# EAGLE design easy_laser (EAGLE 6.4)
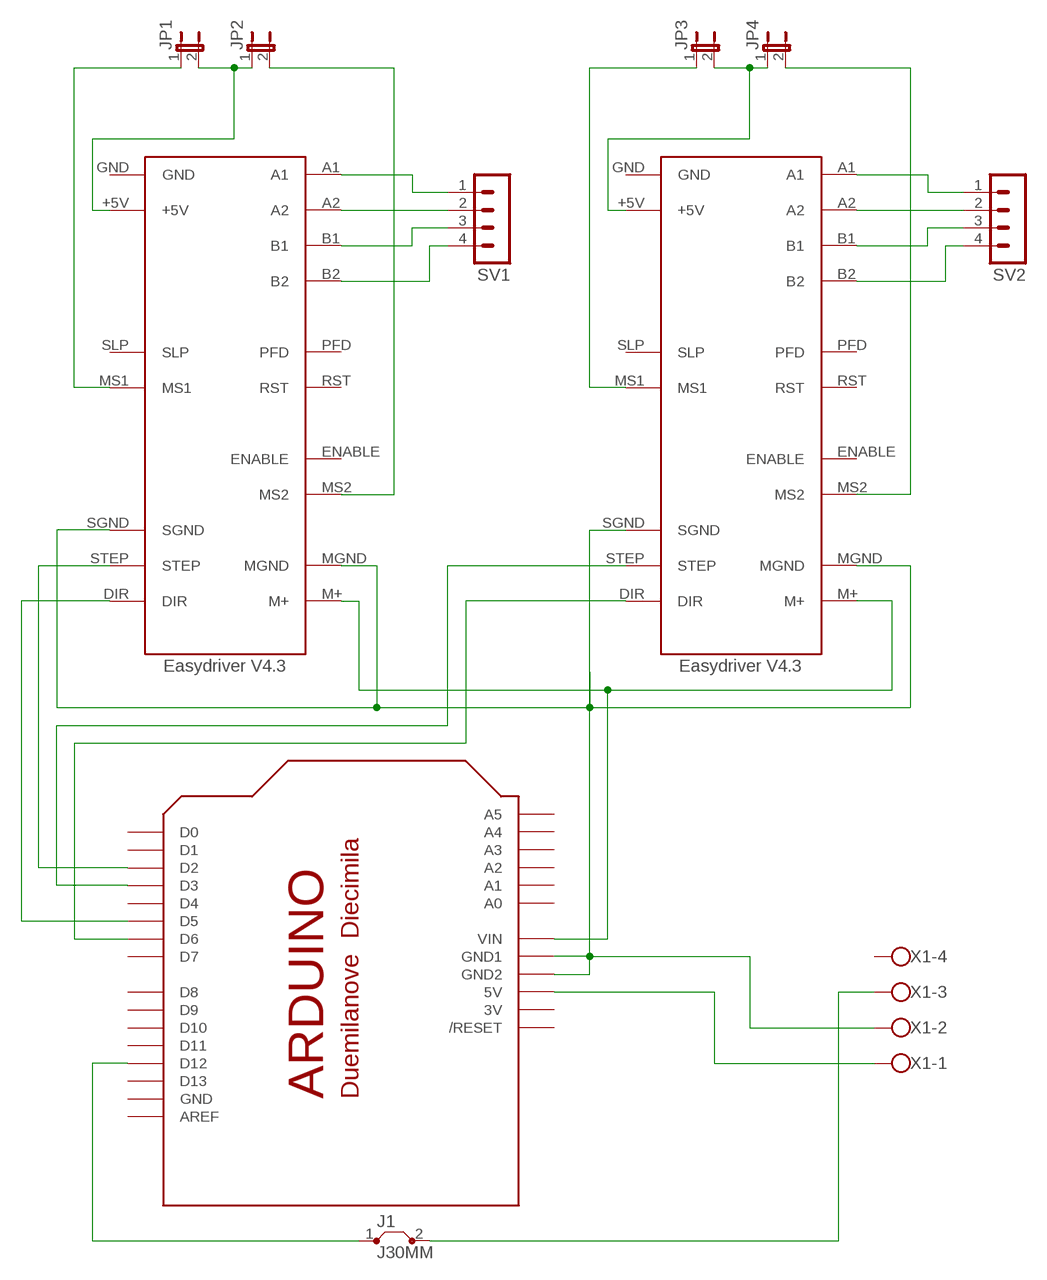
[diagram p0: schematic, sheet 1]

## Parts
J1  J30MM  [30]
JP1  JP1E  [JP1]
JP2  JP1E  [JP1]
JP3  JP1E  [JP1]
JP4  JP1E  [JP1]
SV1  MA04-1  [MA04-1]
SV2  MA04-1  [MA04-1]
U$1  EASYDRIVER  [EASYDRIVER]
U$2  EASYDRIVER  [EASYDRIVER]
U$4  ARDUINO-NOHOLE  [ARDUINO-NOHOLE]
X1  W237-4  [W237-4]

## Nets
N$1: JP3.2 JP4.1 U$2.+5V
N$2: SV1.1 U$1.A1
N$3: U$4.5V X1.1
N$4: JP1.1 U$1.MS1
N$5: JP2.2 U$1.MS2
N$6: JP4.2 U$2.MS2
N$7: U$1.STEP U$4.D2
N$8: U$2.STEP U$4.D3
N$9: U$1.DIR U$4.D5
N$10: U$2.DIR U$4.D6
N$12: JP3.1 U$2.MS1
N$13: SV1.2 U$1.A2
N$14: J1.2 X1.3
N$15: JP1.2 JP2.1 U$1.+5V
N$16: J1.1 U$4.D12
N$17: SV1.3 U$1.B1
N$18: SV1.4 U$1.B2
N$19: SV2.1 U$2.A1
N$20: SV2.2 U$2.A2
N$21: SV2.3 U$2.B1
N$22: SV2.4 U$2.B2
N$28: U$1.MGND U$1.SGND U$2.MGND U$2.SGND U$4.GND1 U$4.GND2 X1.2
N$31: U$1.M+ U$2.M+ U$4.VIN
Unconnected: U$1.ENABLE U$1.PFD U$1.RST U$1.SLP U$2.ENABLE U$2.PFD U$2.RST U$2.SLP U$4.A0 U$4.A1 U$4.A2 U$4.A3 U$4.A4 U$4.A5 U$4.AREF U$4.D0 U$4.D1 U$4.D4 U$4.D7 U$4.D8 U$4.D9 U$4.D10 U$4.D11 U$4.D13 U$4.RESET(/RESET) X1.4

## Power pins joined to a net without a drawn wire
3V: U$4.3V
GND: U$1.GND U$2.GND U$4.GND

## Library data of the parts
J1 = jumper:J: Bridge
JP1-JP4 = jumper:JP1E: JUMPER
SV1 SV2 = con-lstb:MA04-1: PIN HEADER
U$1 U$2 = easydriver:EASYDRIVER: Easydriver V4.3
U$4 = adafruit:ARDUINO: Arduino Diecimila/Duemilanove Make a shield with ease, this package has all the named pins as well as the two mounting drill holes and an outline of the USB and DC power connector. The outline is on the DIMENSION layer, so if your board house uses it they will cut the outline to match.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
X1 = con-wago-500:W237-4: WAGO SCREW CLAMP; OC_FARNELL: unknown; OC_NEWARK: unknown

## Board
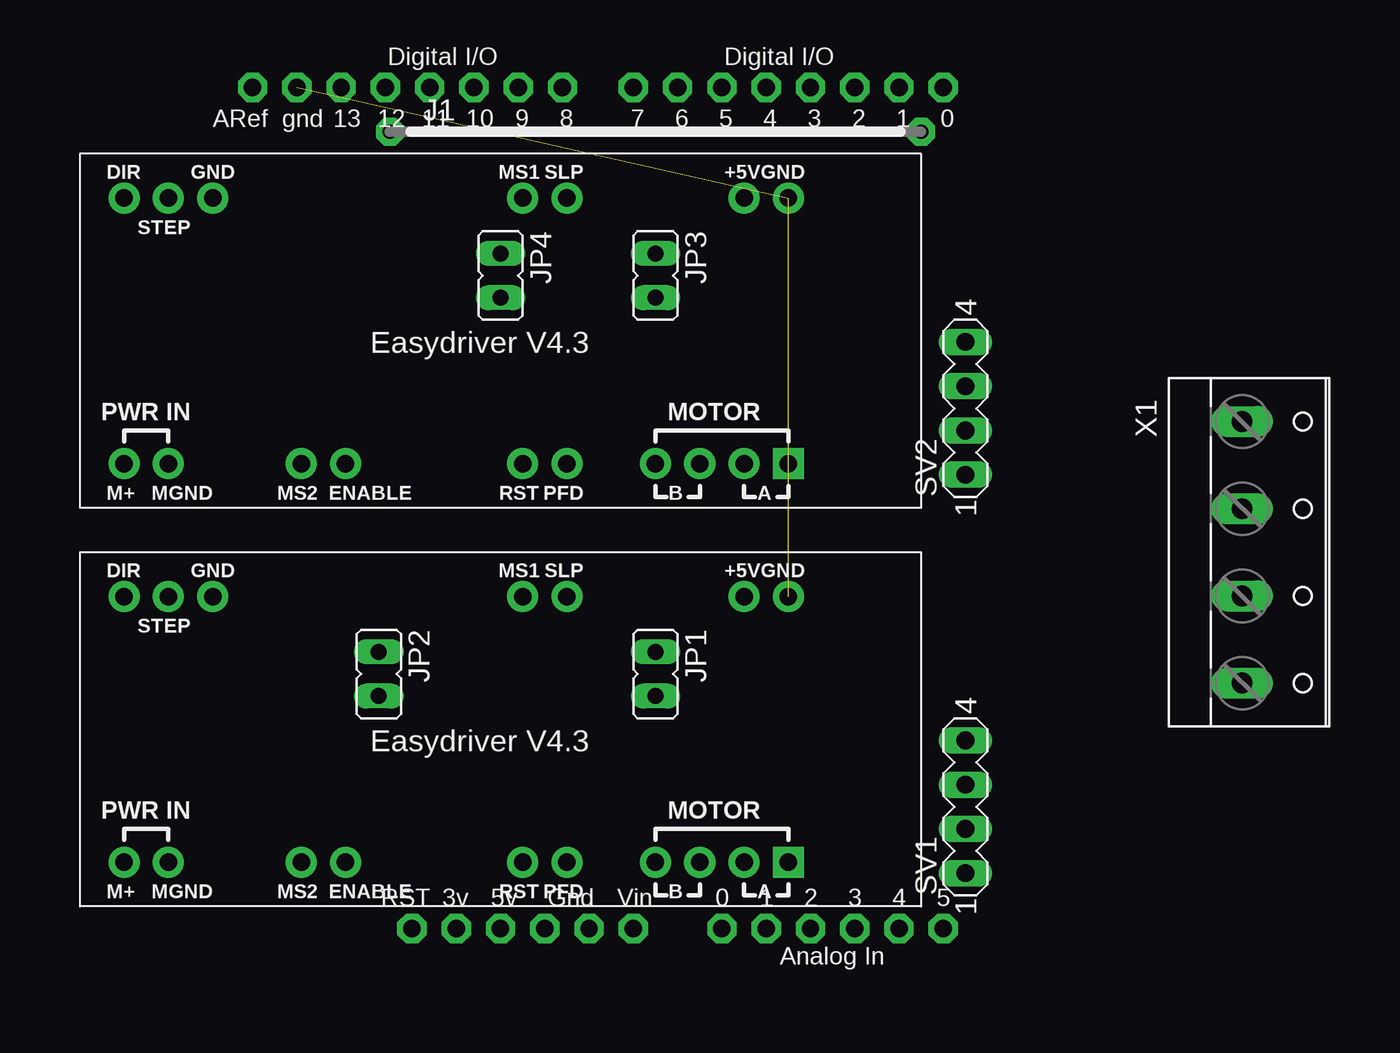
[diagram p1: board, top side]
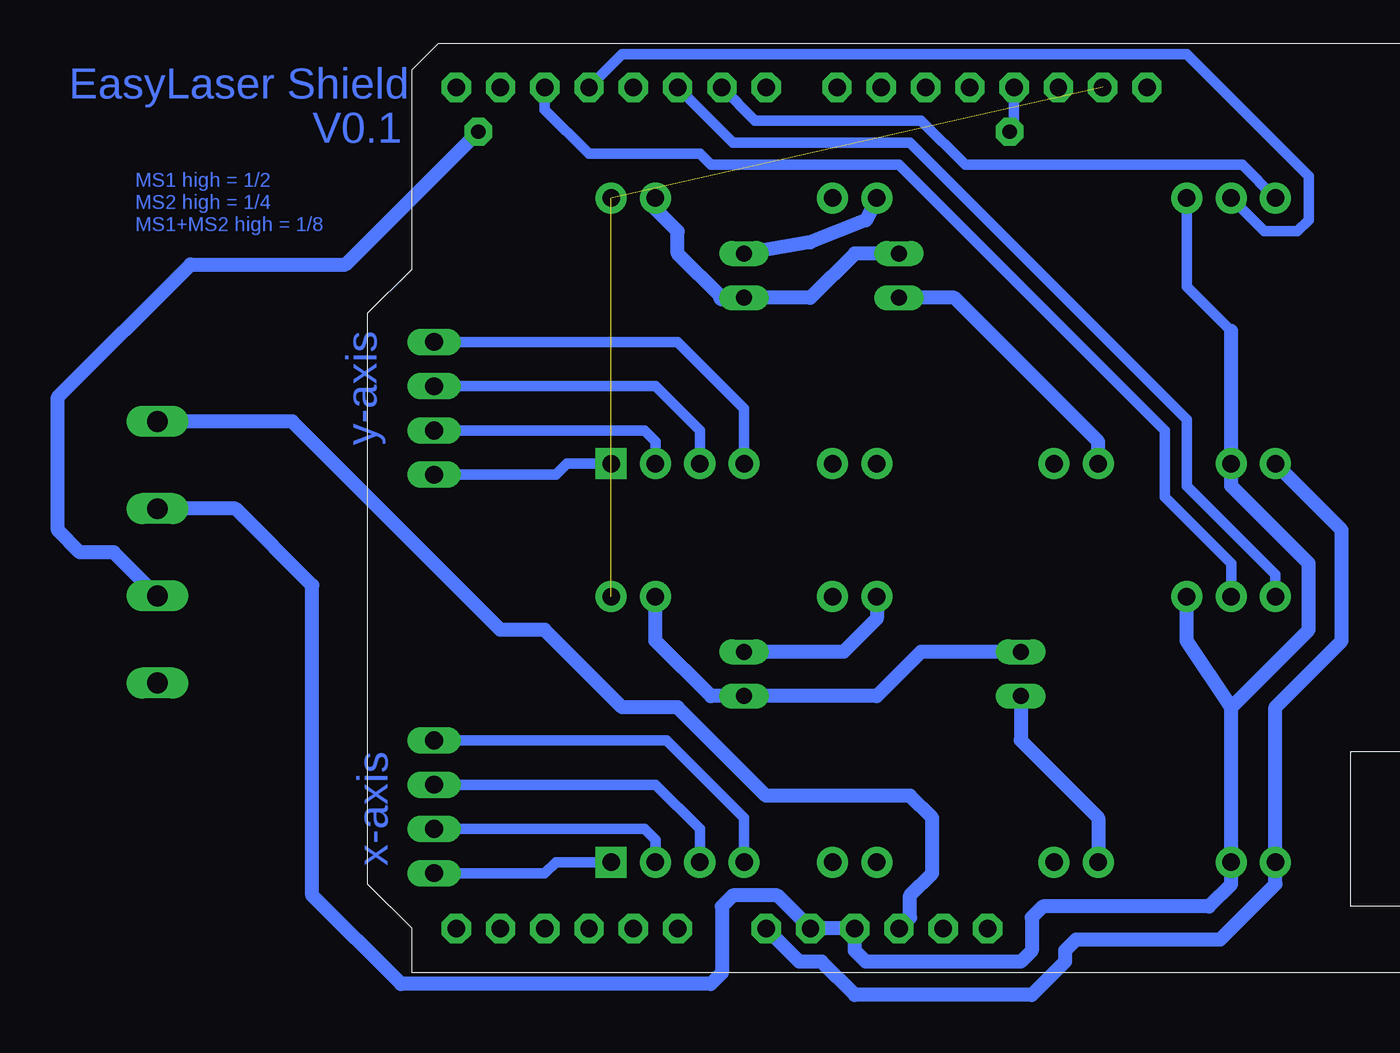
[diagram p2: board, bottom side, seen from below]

No outline drawn. Coordinates in mm, seen from the top.
Copper layers (1*16): Top 0.035mm / dielectric 1.5mm / Bottom 0.035mm
Design rules "default": minimum track width 10mil, minimum drill 24mil, track to track 8mil, track to pad 8mil, pad to pad 8mil, via to via 8mil, smd to smd 8mil, copper to edge 40mil, drill to drill 8mil, minimum pad ring 10mil, minimum via ring 8mil, stop-mask expansion 4mil, vias tented up to drill 0mil, thermal gap 10mil

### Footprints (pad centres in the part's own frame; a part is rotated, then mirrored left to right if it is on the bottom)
30 = drill 0.813 pad 1.6 octagon: 1 -15.24,0; 2 15.24,0
JP1 = drill 0.914 long: 1 0,-1.27; 2 0,1.27
MA04-1 = drill 1.016 long: 1 -3.81,0; 2 -1.27,0; 3 1.27,0; 4 3.81,0
EASYDRIVER = drill 1 pad 1.778: +5V -13.97,-7.62; A2 -13.97,7.62; B1 -11.43,7.62; B2 -8.89,7.62; DIR 21.59,-7.62; ENABLE 8.89,7.62; GND -16.51,-7.62; M+ 21.59,7.62; MGND 19.05,7.62; MS1 -1.27,-7.62; MS2 11.43,7.62; PFD -3.81,7.62; RST -1.27,7.62; SGND 16.51,-7.62; SLP -3.81,-7.62; STEP 19.05,-7.62 | drill 1 pad 1.778 square: A1 -16.51,7.62
ARDUINO-NOHOLE = drill 1 pad 1.676 octagon: 3V 35.56,2.54; 5V 38.1,2.54; A0 50.8,2.54; A1 53.34,2.54; A2 55.88,2.54; A3 58.42,2.54; A4 60.96,2.54; A5 63.5,2.54; AREF 23.876,50.8; D0 63.5,50.8; D1 60.96,50.8; D2 58.42,50.8; D3 55.88,50.8; D4 53.34,50.8; D5 50.8,50.8; D6 48.26,50.8; D7 45.72,50.8; D8 41.656,50.8; D9 39.116,50.8; D10 36.576,50.8; D11 34.036,50.8; D12 31.496,50.8; D13 28.956,50.8; GND 26.416,50.8; GND1 43.18,2.54; GND2 40.64,2.54; RESET 33.02,2.54; VIN 45.72,2.54
W237-4 = drill 1.194 long: 1 -7.5,-1.27; 2 -2.5,-1.27; 3 2.5,-1.27; 4 7.5,-1.27

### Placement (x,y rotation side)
J1  46.99,55.24 0 top
JP1  46.99,24.13 180 top
JP2  31.11,24.13 180 top
JP3  46.99,46.99 180 top
JP4  38.1,46.99 180 top
SV1  64.77,16.51 90 top
SV2  64.77,39.37 90 top
U$1  38.1,20.95 180 top
U$2  38.1,43.81 180 top
U$4  0,6.99 0 top
X1  81.92,31.11 270 top

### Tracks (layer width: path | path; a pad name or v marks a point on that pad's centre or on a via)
GND  (2 unrouted)
N$1
  Bottom 0.813: JP4.1 40.64,48.26 43.18,45.72 JP3.2 | 48.26,45.72 50.8,48.26 50.8,49.53 52.07,50.8 U$2.+5V
  Bottom 1.016: JP3.2 48.26,45.72
N$2
  Bottom 0.61: U$1.A1 57.78,13.34 58.42,12.7 SV1.1
N$3
  Bottom 0.813: U$4.5V 37.47,10.16 37.47,11.43 36.2,12.7 36.2,15.88 37.47,17.14 45.72,17.14 50.8,22.23 53.98,22.23 58.42,26.67 60.96,26.67 72.91,38.62 X1.1
N$4
  Bottom 0.813: U$1.MS1 39.37,27.3 41.27,25.4 JP1.1
N$5
  Bottom 0.813: JP2.2 31.11,20.32 26.67,15.88 U$1.MS2
N$6
  Bottom 0.813: U$2.MS2 26.67,37.47 34.92,45.72 JP4.2
N$7
  Bottom 0.61: U$4.D2 58.42,56.52 55.88,53.98 49.53,53.98 48.9,53.34 38.1,53.34 22.86,38.1 22.86,34.29 19.05,30.48 U$1.STEP
N$8
  Bottom 0.61: U$4.D3 53.98,59.69 21.59,59.69 14.61,52.7 14.61,50.16 15.24,49.53 17.14,49.53 U$2.STEP
N$9
  Bottom 0.61: U$4.D5 47.62,54.61 37.47,54.61 21.59,38.73 21.59,34.92 16.51,29.84 U$1.DIR
N$10
  Bottom 0.61: U$4.D6 46.35,55.88 36.83,55.88 34.29,53.34 18.41,53.34 U$2.DIR
N$12
  Bottom 0.813: U$2.MS1 40.01,50.16 43.18,48.9 JP3.1
N$13
  Bottom 0.61: SV1.2 52.7,15.24 52.07,14.61 U$1.A2
N$14
  Bottom 0.813: X1.3 83.14,31.11 85.09,31.11 86.36,32.38 86.36,40.01 78.74,47.62 69.85,47.62 J1.2
N$15
  Bottom 0.813: JP2.1 36.83,25.4 39.37,22.86 JP1.2 48.9,22.86 52.07,26.04 U$1.+5V
N$16
  Bottom 0.61: J1.1 31.5,55.5 U$4.D12
N$17
  Bottom 0.61: SV1.3 52.07,17.78 49.53,15.24 U$1.B1
N$18
  Bottom 0.61: SV1.4 51.44,20.32 46.99,15.88 U$1.B2
N$19
  Bottom 0.61: SV2.1 57.78,35.56 57.15,36.2 U$2.A1
N$20
  Bottom 0.61: SV2.2 52.7,38.1 52.07,37.47 U$2.A2
N$21
  Bottom 0.61: SV2.3 52.07,40.64 49.53,38.1 U$2.B1
N$22
  Bottom 0.61: SV2.4 50.8,43.18 46.99,39.37 U$2.B2
N$28
  Bottom 0.61: U$2.SGND 21.59,46.35 19.05,43.81
  Bottom 0.813: 19.05,43.81 U$2.MGND 19.05,34.92 14.61,30.48 14.61,26.67 19.05,22.23 | U$1.SGND 21.59,26.04 19.05,22.23 | 19.05,22.23 U$1.MGND 19.05,12.06 20.32,10.79 29.84,10.79 30.48,10.16 30.48,8.26 31.11,7.62 40.01,7.62 40.64,8.26 U$4.GND2 U$4.GND1 45.09,11.43 47.62,11.43 48.26,10.79 48.26,6.99 48.9,6.35 66.67,6.35 71.75,11.43 71.75,29.21 76.16,33.62 X1.2
N$31
  Bottom 0.813: U$2.M+ 12.7,32.38 12.7,26.04 16.51,22.23 U$1.M+ 16.51,12.06 19.68,8.89 27.94,8.89 28.57,8.26 28.57,7.62 30.48,5.71 40.64,5.71 42.55,7.62 43.81,7.62 U$4.VIN

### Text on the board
Bottom: EasyLaser Shield | V0.1 | MS1 high = 1/2 | MS2 high = 1/4 | MS1+MS2 high = 1/8 | y-axis | x-axis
